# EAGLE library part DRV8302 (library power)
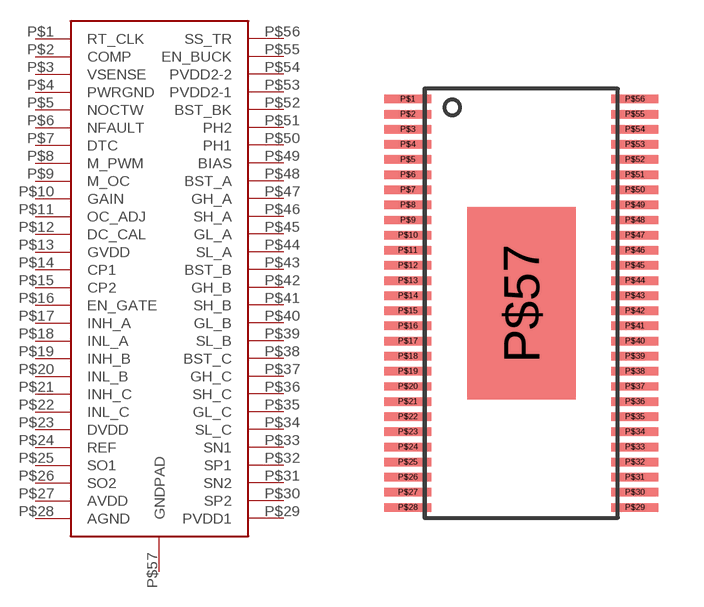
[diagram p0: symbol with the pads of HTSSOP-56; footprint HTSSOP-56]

Designator prefix U

## DRV8302  [HTSSOP-56]
P$1  RT_CLK
P$2  COMP
P$3  VSENSE
P$4  PWRGND
P$5  NOCTW
P$6  NFAULT
P$7  DTC
P$8  M_PWM
P$9  M_OC
P$10  GAIN
P$11  OC_ADJ
P$12  DC_CAL
P$13  GVDD
P$14  CP1
P$15  CP2
P$16  EN_GATE
P$17  INH_A
P$18  INL_A
P$19  INH_B
P$20  INL_B
P$21  INH_C
P$22  INL_C
P$23  DVDD
P$24  REF
P$25  SO1
P$26  SO2
P$27  AVDD
P$28  AGND
P$29  PVDD1
P$30  SP2
P$31  SN2
P$32  SP1
P$33  SN1
P$34  SL_C
P$35  GL_C
P$36  SH_C
P$37  GH_C
P$38  BST_C
P$39  SL_B
P$40  GL_B
P$41  SH_B
P$42  GH_B
P$43  BST_B
P$44  SL_A
P$45  GL_A
P$46  SH_A
P$47  GH_A
P$48  BST_A
P$49  BIAS
P$50  PH1
P$51  PH2
P$52  BST_BK
P$53  PVDD2-1
P$54  PVDD2-2
P$55  EN_BUCK
P$56  SS_TR
P$57  GNDPAD

## Footprint HTSSOP-56 (pad centres in mm)
smd 1.549 x 0.279: P$1 -3.75,6.75; P$2 -3.75,6.25; P$3 -3.75,5.75; P$4 -3.75,5.25; P$5 -3.75,4.75; P$6 -3.75,4.25; P$7 -3.75,3.75; P$8 -3.75,3.25; P$9 -3.75,2.75; P$10 -3.75,2.25; P$11 -3.75,1.75; P$12 -3.75,1.25; P$13 -3.75,0.75; P$14 -3.75,0.25; P$15 -3.75,-0.25; P$16 -3.75,-0.75; P$17 -3.75,-1.25; P$18 -3.75,-1.75; P$19 -3.75,-2.25; P$20 -3.75,-2.75; P$21 -3.75,-3.25; P$22 -3.75,-3.75; P$23 -3.75,-4.25; P$24 -3.75,-4.75; P$25 -3.75,-5.25; P$26 -3.75,-5.75; P$27 -3.75,-6.25; P$28 -3.75,-6.75; P$29 3.75,-6.75; P$30 3.75,-6.25; P$31 3.75,-5.75; P$32 3.75,-5.25; P$33 3.75,-4.75; P$34 3.75,-4.25; P$35 3.75,-3.75; P$36 3.75,-3.25; P$37 3.75,-2.75; P$38 3.75,-2.25; P$39 3.75,-1.75; P$40 3.75,-1.25; P$41 3.75,-0.75; P$42 3.75,-0.25; P$43 3.75,0.25; P$44 3.75,0.75; P$45 3.75,1.25; P$46 3.75,1.75; P$47 3.75,2.25; P$48 3.75,2.75; P$49 3.75,3.25; P$50 3.75,3.75; P$51 3.75,4.25; P$52 3.75,4.75; P$53 3.75,5.25; P$54 3.75,5.75; P$55 3.75,6.25; P$56 3.75,6.75
smd 3.581 x 6.35: P$57 0,0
